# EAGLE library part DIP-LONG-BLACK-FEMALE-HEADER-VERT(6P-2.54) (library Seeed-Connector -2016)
320030012
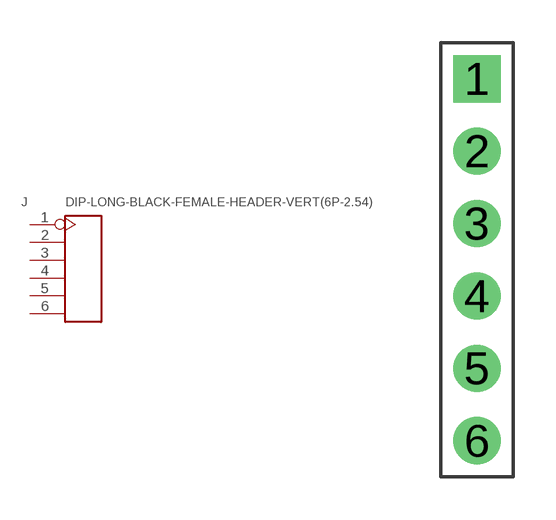
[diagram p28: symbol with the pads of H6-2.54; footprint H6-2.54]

Designator prefix J

## DIP-LONG-BLACK-FEMALE-HEADER-VERT(6P-2.54) (MPN: F185-1106A1BSYA2; VALUE: 6p-2.54)  [H6-2.54]
1  1
2  2
3  3
4  4
5  5
6  6

## Footprint H6-2.54 (pad centres in mm)
drill 0.889 pad 1.651 square: 1 0,6.35
drill 0.889 pad 1.651: 2 0,3.81; 3 0,1.27; 4 0,-1.27; 5 0,-3.81; 6 0,-6.35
